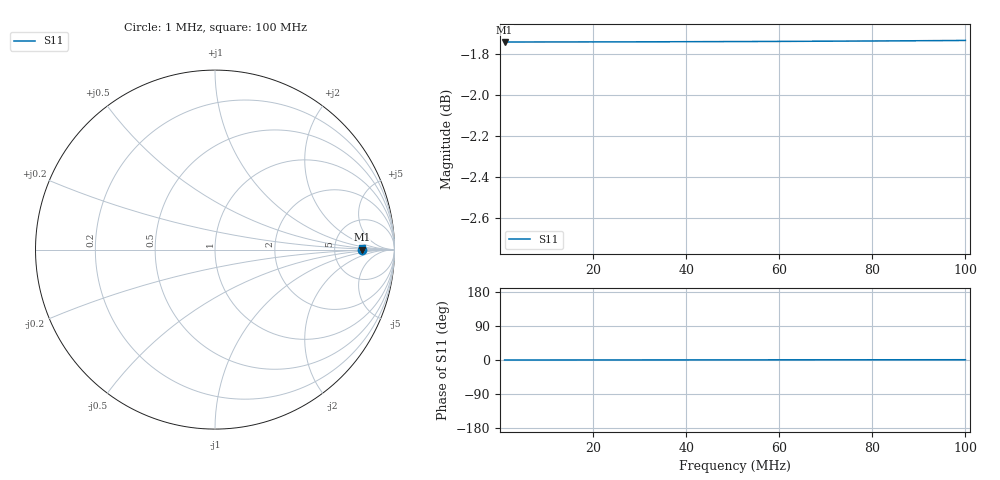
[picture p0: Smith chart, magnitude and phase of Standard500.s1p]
# MHz S RI R 50.0
! SimSmith 18.4g
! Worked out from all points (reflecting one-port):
!   1000 points, 1 MHz to 100 MHz, reference 50 ohm
!   lowest |S11| = -1.7 dB at 1 MHz (marker M1), VSWR 10.00, Z = 500 + j0.314 ohm
!   phase of S11 starts at 0 deg and turns +1 deg over the sweep
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1  0.8182 0.000104
1.198198  0.8182 0.000124
1.297297  0.8182 0.000135
1.495496  0.8182 0.000155
7.342342  0.8182 0.000762
13.38739  0.8182 0.00139
19.53153  0.8182 0.00203
22.6036  0.8182 0.00235
25.77478  0.8182 0.00268
28.84685  0.8182 0.00299
32.01802  0.8183 0.00332
38.16216  0.8183 0.00396
41.33333  0.8183 0.00429
44.40541  0.8183 0.00461
50.54955  0.8184 0.00524
56.69369  0.8184 0.00588
59.76577  0.8184 0.0062
62.93694  0.8184 0.00653
66.00901  0.8185 0.00684
69.18018  0.8185 0.00717
75.32432  0.8186 0.0078
81.46847  0.8186 0.00844
87.71171  0.8187 0.00908
93.55856  0.8187 0.00968
99.5045  0.8188 0.0103
99.7027  0.8188 0.0103
99.9009  0.8188 0.0103
100  0.8188 0.0103
